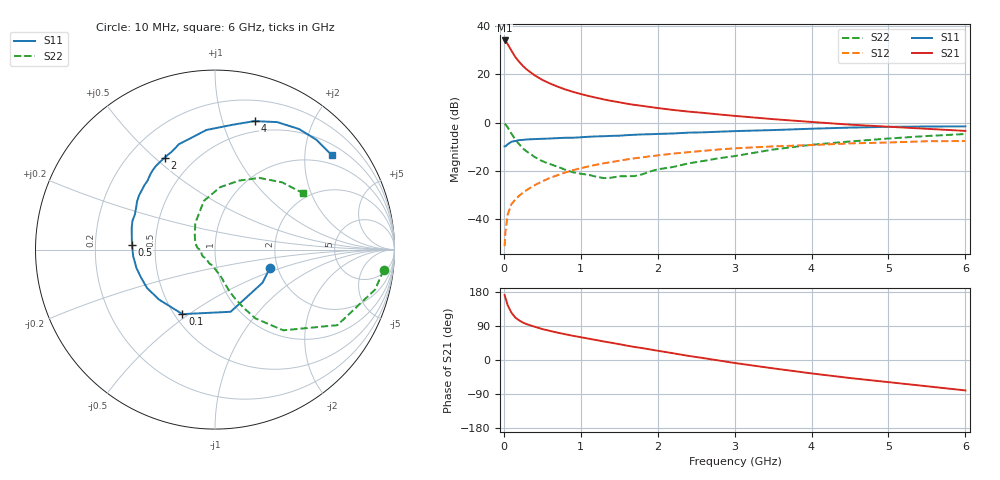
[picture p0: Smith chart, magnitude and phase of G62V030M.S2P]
! SIEMENS Small Signal Semiconductors
! BFG193
! Si NPN RF Bipolar Junction Transistor in SOT223
! VCE = 2 V  IC = 30 mA
! Common Emitter S-Parameters:  August  1996
# GHz  S  MA  R  50
!  f  S11  S21  S12  S22
! GHz  MAG  ANG  MAG  ANG  MAG  ANG  MAG  ANG
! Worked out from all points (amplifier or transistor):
!   36 points, 10 MHz to 6 GHz, reference 50 ohm
!   highest |S21| = 34.0 dB at 10 MHz (marker M1)
!   |S21| within 3 dB of that: start of sweep to 76.74 MHz
!   unconditionally stable (mu >= 1): 510.6 MHz to 2.615 GHz
!   at 250 MHz: K = 0.85, MSG = 26.1 dB, |S12| = -28.9 dB
!   at 1.4 GHz: K = 1.05, MAG = 11.3 dB, |S12| = -16.3 dB
!   at 6 GHz: K = 0.92, MSG = 2.1 dB, |S12| = -7.6 dB
!   S11 on the Smith chart (normalised r, x): 10 MHz: 1.82, -0.41; 100 MHz: 0.55, -0.47; 500 MHz: 0.37, +0.03; 2 GHz: 0.35, +0.54; 4 GHz: 0.39, +1.28; 6 GHz: 0.75, +2.64
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0.01  0.323 -18.3  49.96 171.7  0.0028 85.6  0.9462 -6.9
0.02  0.3227 -35.0  48.7 164.6  0.0054 79.5  0.9196 -14.0
0.05  0.3572 -75.9  41.9 144.5  0.0126 66.5  0.8012 -31.7
0.1  0.4028 -116.8  30.52 124.5  0.0208 62.9  0.5888 -49.8
0.15  0.4182 -138.3  22.66 111.7  0.0258 59.9  0.4442 -59.6
0.2  0.4349 -150.6  18.01 104.5  0.031 61.2  0.3564 -64.1
0.25  0.4405 -159.3  14.72 98.6  0.0358 62.1  0.2917 -67.9
0.3  0.4494 -166.6  12.47 94.3  0.0408 63.1  0.2523 -70.5
0.4  0.4575 -175.6  9.524 87.8  0.0509 64.1  0.1954 -74.1
0.5  0.4636 176.6  7.656 81.7  0.0612 63.5  0.16 -76.8
0.6  0.4699 170.6  6.437 76.8  0.0722 63.1  0.1391 -80.2
0.8  0.4869 160.9  4.847 67.9  0.0934 60.5  0.1063 -90.3
1.1  0.5104 148.3  3.558 56.4  0.1246 55.7  0.0836 -111.9
1.6  0.5519 130.9  2.46 37.9  0.1737 45.0  0.0782 -160.9
2  0.5845 118.7  2.004 24.5  0.2106 36.0  0.1083 166.2
2.2  0.5973 113.6  1.83 17.8  0.2289 31.4  0.1213 155.5
2.8  0.6498 98.2  1.476 -1.5  0.2796 17.3  0.1844 126.7
3.5  0.7023 82.0  1.182 -22.0  0.3229 0.0  0.2782 102.9
4  0.7491 72.9  1.033 -35.4  0.3446 -9.8  0.349 85.3
4.5  0.7903 64.0  0.909 -47.6  0.3725 -19.9  0.4081 70.5
5.5  0.8328 47.3  0.746 -69.3  0.4128 -42.8  0.5295 45.0
6  0.837 39.0  0.675 -80.3  0.4163 -56.0  0.5825 32.7
